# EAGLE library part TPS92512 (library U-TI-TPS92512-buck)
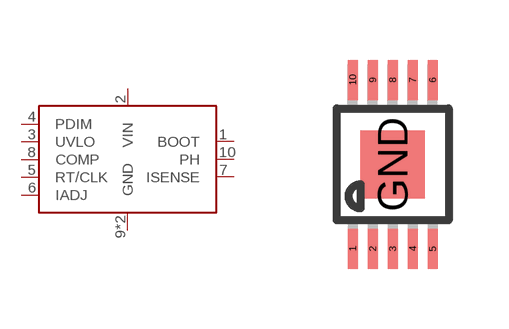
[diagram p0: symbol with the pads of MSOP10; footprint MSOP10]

Designator prefix -

## TPS92512  [MSOP10]
1  BOOT
2  VIN
3  UVLO
4  PDIM
5  RT/CLK
6  IADJ
7  ISENSE
8  COMP
9  GND
10  PH
GND  GND

## Footprint MSOP10 (pad centres in mm)
10-Lead Mini Small Outline Package [MSOP] (RM-10) Source: http://www.analog.com/UploadedFiles/Data_Sheets/35641221898805SSM2167_b.pdf COMPLIANT TO JEDEC STANDARDS MO-187BA
smd 0.25 x 1: 1 -1,-2.113; 2 -0.5,-2.113; 3 0,-2.113; 4 0.5,-2.113; 5 1,-2.113; 6 1,2.113; 7 0.5,2.113; 8 0,2.113; 9 -0.5,2.113; 10 -1,2.113
smd 1.6 x 1.7: GND 0,0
